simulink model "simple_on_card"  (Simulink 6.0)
settings: Solver=ode45  StartTime=0.0  StopTime=10.0  RelTol=1e-3
libraries: ADlibrary x3

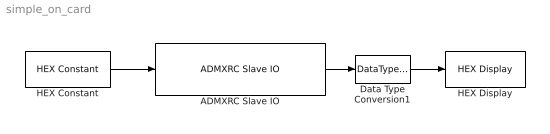
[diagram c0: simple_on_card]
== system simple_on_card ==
  ADMXRC Slave IO : ADlibrary/Hardware in the Loop/ADMXRC Slave IO  filename=g:\tmp2\simple.bit  clock_freq=33  input_width=1  output_width=1  tll=1000  index=0
  Data Type Conversion1 : DataTypeConversion  OutDataTypeMode=double
  HEX Constant : ADlibrary/Miscellaneous/HEX Constant  value=1234abcd
  HEX Display : ADlibrary/Miscellaneous/HEX Display
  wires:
  HEX Constant/1 -> ADMXRC Slave IO/1
  Data Type Conversion1/1 -> HEX Display/1
  ADMXRC Slave IO/1 -> Data Type Conversion1/1
